FUNCTION_BLOCK FB_DO_IED_LD1_XCBR1_BlkOpn EXTENDS FB_AcsiCommonControllableDataClass
VAR_INPUT
	stVal: FB_AcsiBATypeBOOLEAN := (fc:=ACSI_FC_ST, TrgOp:=ACSI_TrgOp_dchg, bLinkResult:=THIS^.AddDataToContainer(ipData:=stVal));
	q: FB_AcsiDATypeQuality := (fc:=ACSI_FC_ST, TrgOp:=ACSI_TrgOp_qchg, bLinkResult:=THIS^.AddDataToContainer(ipData:=q));
	t: FB_AcsiDATypeTimeStamp := (fc:=ACSI_FC_ST, bLinkResult:=THIS^.AddDataToContainer(ipData:=t));
	ctlModel: FB_AcsiDATypeCtlModels := (fc:=ACSI_FC_CF, TrgOp:=ACSI_TrgOp_dchg, eValue:=E_AcsiCtlModels.StatusOnly, bLinkResult:=THIS^.AddDataToContainer(ipData:=ctlModel));
END_VAR
VAR
END_VAR

END_FUNCTION_BLOCK
